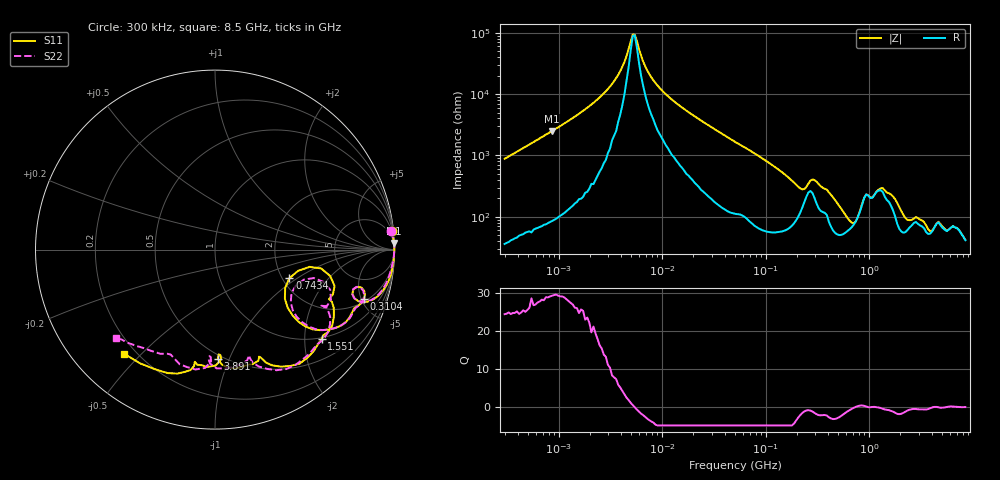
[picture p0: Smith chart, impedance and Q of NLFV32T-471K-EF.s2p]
! S-parameter Generated by TDK Corporation
! Copyright(C) 2015 TDK Corporation.
! All Rights Reserved.
! TDK P/N: NLFV32T-471K-EF (Inductors)
! Property: L=470uH at 796kHz
! Size(LxWxT): 3.2x2.5x2.2mm, 0.126x0.098x0.087inches
! Model Type: s2p (Touchstone File Format Version 1.0)
! Frequency: DC=Yes Start=0.3MHz Stop=8500MHz 225points Log-sweep
! Note:
! Model Generated on Jun. 23, 2015
! Hash(MD5):
! Port Assignments:
!  1 ---@@@--- 2
! Applicable Conditions:
!  Temperature = 25 degC
!  DC Bias Current = 0 A
!  Small Signal Operation
! Terms and conditions regarding TDK Simulation Models
! (1)This simulation model is being provided solely for informational purposes. Please refer to the specifications of the products in terms of detailed characteristics of such products.
! (2)In no event shall TDK Corporation of any of its subsidiaries be liable for any loss or damage arising, directly or indirectly,
!  From any information contained in this simulation model, including, but not limited to loss or damages arising from any inaccuracies, omissions or errors in connection with such information.
! (3)Any and all copyrights on this simulation model are owned by TDK Corporation.
!  Duplication or redistribution of this simulation model without prior written permission from TDK Corporation is prohibited.
! (4)This simulation model is subject to any modification or change without any prior notice.
! (5)Neither TDK Corporation nor any of its subsidiaries shall make any warranty, express or implied,
!  Including but not limited to the correctness, implied warranties of merchantability and fitness for a particular purpose with respect to this simulation models.
! (6)The use of this simulation model shall be deemed to have consented to the terms and conditions hereof.
# MHz S MA R 50
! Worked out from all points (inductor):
!   224 points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, 300 kHz to 8.5 GHz, reference 50 ohm
!   read as one part in series: L = 461 uH near 314.1 kHz
!   highest Q = 29.2 at 863.6 kHz (marker M1), where L = 460 uH
!   self-resonance near 5.188 MHz
!   S11 on the Smith chart (normalised r, x): 300 kHz: 2, +19; 310.4 MHz: 2.26, -5.28; 743.4 MHz: 2.18, -0.87; 1.551 GHz: 0.96, -2.41; 3.891 GHz: 0.47, -0.91; 8.5 GHz: 0.16, -0.45
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0.3  0.9895 6.1  0.1124 -81.6  0.1139 -81.8  0.9887 6.1
0.8636283  0.9975 2.1  0.03991 -85.9  0.04012 -86.3  0.9975 2.1
1.72111  0.9989 1.0  0.01873 -86.8  0.01878 -87.2  0.9993 0.9
3.591337  0.9992 0.2  0.005479 -82.0  0.005489 -82.3  0.9993 0.1
4.316363  0.9991 0.0  0.002979 -72.8  0.002984 -73.2  0.9991 -0.1
5.187759  0.999 -0.1  0.001067 -20.5  0.001061 -21.5  0.999 -0.2
7.157115  0.9987 -0.4  0.00408 72.1  0.004085 71.7  0.9988 -0.5
9.430415  0.9986 -0.7  0.007925 79.0  0.007919 78.8  0.9985 -0.8
51.67171  0.9951 -4.5  0.06104 81.5  0.06106 81.2  0.9921 -4.7
135.6836  0.9714 -12.4  0.1679 71.9  0.168 71.7  0.9648 -12.5
214.8731  0.8496 -19.8  0.2873 47.2  0.2875 46.9  0.8474 -19.7
283.1228  0.8611 -15.3  0.2089 38.3  0.2091 38.1  0.8566 -15.5
310.3886  0.8748 -18.3  0.2316 46.0  0.2317 45.7  0.8722 -18.3
538.8791  0.7022 -39.2  0.4922 30.5  0.4922 30.2  0.7147 -38.3
743.4462  0.444 -21.0  0.5312 -9.0  0.5313 -9.3  0.4932 -23.8
935.5712  0.6963 -16.9  0.2934 -16.0  0.2936 -16.5  0.7037 -23.4
1551.304  0.7764 -40.1  0.2783 5.6  0.2786 5.0  0.7787 -45.0
2240.89  0.691 -65.7  0.4724 -4.8  0.4729 -5.1  0.6634 -71.6
3890.506  0.608 -88.5  0.4841 -37.3  0.4851 -37.8  0.6126 -93.3
4465.833  0.6121 -86.8  0.4108 -51.9  0.4108 -52.3  0.6226 -92.0
6450.987  0.6857 -101.6  0.3369 -70.4  0.3384 -70.5  0.6551 -117.5
8500  0.7696 -131.0  0.2836 -79.7  0.2829 -79.0  0.7384 -138.2
